| TEXAS INSTRUMENTS INCORPORATED
| Standard Linear and Logic Group
| IBIS Model of SN74CBT3383
| 10-BIT FET BUS-EXCHANGE SWITCHES
| This file contains package information for the following:
|  SSOP 24-pin (DB) package as [Component] CBT3383_DB
|  SSOP 24-pin (DBQ) package as [Component] CBT3383_DBQ
|  TVSOP 24-pin (DGV) package as [Component] CBT3383_DGV
|  SOIC 24-pin (DW) package as [Component] CBT3383_DW
|  TSSOP 24-pin (PW) package as [Component] CBT3383_PW
| This device can be powered at the following Vccs:
|  5 volt Vcc
| This file provides unique models under the [Model Selector] for each Vcc.
| For operation at a specific Vcc, select the appropriate model after each
| [Model Selector] keyword.
[IBIS Ver]   3.2
[Comment char]  |_char
[File Name]   sn74cbt3383.ibs
[File Rev]   1.1 | e_die
[Date]   April 17, 2003
[Source]   Data created from TI-SPICE simulations at TI-SLL.
[Notes]   The following is an IBIS list for the CBT3383.
   Please contact sllibis@ti.com with questions and
   comments concerning SLL IBIS models.
   - Power-clamp data has been deleted since there is no
   power-clamp diode in the device.
   - Non-monotonic data due to device characteristics.
[Disclaimer] Property of Texas Instruments Incorporated.  Unauthorized
   reproduction and/or distribution is strictly prohibited.
   This product is protected under copyright law.
   Created  2003, (C) Copyright  2003, Texas Instruments
   Incorporated, All Rights Reserved
   UNLESS THERE IS A SIGNED, WRITTEN AGREEMENT TO THE
   CONTRARY, TEXAS INSTRUMENTS (TI) IS PROVIDING THE IBIS
   MODELS  AND WITHOUT ANY WARRANTY, EXPRESSED OR
   IMPLIED.  TI assumes no liability for:
   1) the accuracy of the IBIS models provided to your
   company;
   2) the proper functioning of these IBIS Models in your
   design or for any resulting applications; or
   3) infringement of patents, copyrights or intellectual
   property rights resulting from your use of these IBIS
   models.
   TI provides IBIS Models as a service to our customers.
   You and your company shall not distribute, sell or give
   these models to anyone else without prior written
   permission from TI.
   TI reserves the right to make changes to our products or
   to discontinue any semiconductor product or service
   without notice, and advises our customers to obtain the
   latest version of relevant information to verify, before
   placing orders, that the information being relied on is
   current.
   Please be aware that your receipt and use of the IBIS
   information provided shall serve as acceptance of these
   terms and conditions.  If you do not accept these terms,
   you should return or destroy the IBIS models and any
   other accompanying information immediately.
| Component CBT3383_DB 24-pin SSOP
[Component]   CBT3383_DB
[Manufacturer]   Texas Instruments, Inc.
[Package]
|   typ   min   max
R_pkg   4.500e-02   4.000e-02   4.900e-02
L_pkg   3.668e-09   3.226e-09   4.415e-09
C_pkg   4.160e-13   3.490e-13   5.070e-13
[Pin]   signal_name   model_name   R_pin   L_pin   C_pin
1   NBE   CBT3383E_NBE   4.200e-02   4.299e-09   5.030e-13
2   1B1   CBT3383E_IO   4.000e-02   3.960e-09   4.990e-13
3   1A1   CBT3383E_IO   4.200e-02   3.775e-09   4.170e-13
4   1A2   CBT3383E_IO   4.700e-02   3.487e-09   3.690e-13
5   1B2   CBT3383E_IO   4.600e-02   3.347e-09   3.520e-13
6   2B1   CBT3383E_IO   4.900e-02   3.352e-09   3.710e-13
7   2A1   CBT3383E_IO   4.600e-02   3.226e-09   3.630e-13
8   2A2   CBT3383E_IO   4.700e-02   3.289e-09   3.490e-13
9   2B2   CBT3383E_IO   4.700e-02   3.347e-09   3.610e-13
10   3B1   CBT3383E_IO   4.100e-02   3.576e-09   4.090e-13
11   3A1   CBT3383E_IO   4.100e-02   3.995e-09   5.030e-13
12   GND   GND   4.500e-02   4.415e-09   5.070e-13
13   BX   CBT3383E_BX   4.300e-02   4.337e-09   5.060e-13
14   3A2   CBT3383E_IO   4.200e-02   4.003e-09   5.040e-13
15   3B2   CBT3383E_IO   4.100e-02   3.686e-09   4.100e-13
16   4B1   CBT3383E_IO   4.800e-02   3.355e-09   3.490e-13
17   4A1   CBT3383E_IO   4.700e-02   3.301e-09   3.530e-13
18   4A2   CBT3383E_IO   4.800e-02   3.268e-09   3.660e-13
19   4B2   CBT3383E_IO   4.800e-02   3.269e-09   3.660e-13
20   5B1   CBT3383E_IO   4.700e-02   3.314e-09   3.490e-13
21   5A1   CBT3383E_IO   4.800e-02   3.399e-09   3.550e-13
22   5A2   CBT3383E_IO   4.100e-02   3.688e-09   4.120e-13
23   5B2   CBT3383E_IO   4.200e-02   4.003e-09   5.040e-13
24   VCC   POWER   4.300e-02   4.347e-09   5.050e-13
| Component CBT3383_DBQ 24-pin SSOP
[Component]   CBT3383_DBQ
[Manufacturer]   Texas Instruments, Inc.
[Package]
|   typ   min   max
R_pkg   4.400e-02   3.100e-02   6.600e-02
L_pkg   3.074e-09   2.348e-09   4.044e-09
C_pkg   3.220e-13   2.340e-13   4.460e-13
[Pin]   signal_name   model_name   R_pin   L_pin   C_pin
1   NBE   CBT3383E_NBE   6.500e-02   4.044e-09   4.290e-13
2   1B1   CBT3383E_IO   6.600e-02   3.824e-09   4.460e-13
3   1A1   CBT3383E_IO   3.100e-02   3.011e-09   3.210e-13
4   1A2   CBT3383E_IO   3.200e-02   2.699e-09   2.590e-13
5   1B2   CBT3383E_IO   3.500e-02   2.519e-09   2.450e-13
6   2B1   CBT3383E_IO   3.500e-02   2.348e-09   2.340e-13
7   2A1   CBT3383E_IO   3.500e-02   2.348e-09   2.340e-13
8   2A2   CBT3383E_IO   3.500e-02   2.518e-09   2.450e-13
9   2B2   CBT3383E_IO   3.200e-02   2.699e-09   2.590e-13
10   3B1   CBT3383E_IO   3.100e-02   3.011e-09   3.210e-13
11   3A1   CBT3383E_IO   6.600e-02   3.824e-09   4.460e-13
12   GND   GND   6.500e-02   4.044e-09   4.290e-13
13   BX   CBT3383E_BX   6.500e-02   4.044e-09   4.290e-13
14   3A2   CBT3383E_IO   6.600e-02   3.824e-09   4.460e-13
15   3B2   CBT3383E_IO   3.100e-02   3.011e-09   3.210e-13
16   4B1   CBT3383E_IO   3.200e-02   2.699e-09   2.590e-13
17   4A1   CBT3383E_IO   3.500e-02   2.518e-09   2.450e-13
18   4A2   CBT3383E_IO   3.500e-02   2.348e-09   2.340e-13
19   4B2   CBT3383E_IO   3.500e-02   2.348e-09   2.340e-13
20   5B1   CBT3383E_IO   3.500e-02   2.518e-09   2.450e-13
21   5A1   CBT3383E_IO   3.200e-02   2.699e-09   2.590e-13
22   5A2   CBT3383E_IO   3.100e-02   3.011e-09   3.210e-13
23   5B2   CBT3383E_IO   6.600e-02   3.824e-09   4.460e-13
24   VCC   POWER   6.500e-02   4.044e-09   4.290e-13
| Component CBT3383_DGV 24-pin TVSOP
[Component]   CBT3383_DGV
[Manufacturer]   Texas Instruments, Inc.
[Package]
|   typ   min   max
R_pkg   4.300e-02   3.900e-02   4.700e-02
L_pkg   2.601e-09   2.312e-09   3.626e-09
C_pkg   3.580e-13   2.770e-13   5.950e-13
[Pin]   signal_name   model_name   R_pin   L_pin   C_pin
1   NBE   CBT3383E_NBE   4.300e-02   3.625e-09   5.950e-13
2   1B1   CBT3383E_IO   4.000e-02   2.656e-09   4.020e-13
3   1A1   CBT3383E_IO   3.900e-02   2.338e-09   3.080e-13
4   1A2   CBT3383E_IO   4.600e-02   2.354e-09   2.770e-13
5   1B2   CBT3383E_IO   4.500e-02   2.312e-09   2.850e-13
6   2B1   CBT3383E_IO   4.700e-02   2.318e-09   2.820e-13
7   2A1   CBT3383E_IO   4.700e-02   2.318e-09   2.820e-13
8   2A2   CBT3383E_IO   4.500e-02   2.312e-09   2.850e-13
9   2B2   CBT3383E_IO   4.600e-02   2.353e-09   2.780e-13
10   3B1   CBT3383E_IO   3.900e-02   2.338e-09   3.080e-13
11   3A1   CBT3383E_IO   4.100e-02   2.660e-09   4.020e-13
12   GND   GND   4.300e-02   3.625e-09   5.950e-13
13   BX   CBT3383E_BX   4.400e-02   3.626e-09   5.940e-13
14   3A2   CBT3383E_IO   4.000e-02   2.658e-09   4.020e-13
15   3B2   CBT3383E_IO   3.900e-02   2.343e-09   3.110e-13
16   4B1   CBT3383E_IO   4.600e-02   2.353e-09   2.780e-13
17   4A1   CBT3383E_IO   4.500e-02   2.312e-09   2.850e-13
18   4A2   CBT3383E_IO   4.700e-02   2.319e-09   2.820e-13
19   4B2   CBT3383E_IO   4.700e-02   2.319e-09   2.820e-13
20   5B1   CBT3383E_IO   4.500e-02   2.312e-09   2.850e-13
21   5A1   CBT3383E_IO   4.600e-02   2.353e-09   2.780e-13
22   5A2   CBT3383E_IO   3.900e-02   2.337e-09   3.080e-13
23   5B2   CBT3383E_IO   4.000e-02   2.658e-09   4.020e-13
24   VCC   POWER   4.400e-02   3.626e-09   5.950e-13
| Component CBT3383_DW 24-pin SOIC
[Component]   CBT3383_DW
[Manufacturer]   Texas Instruments, Inc.
[Package]
|   typ   min   max
R_pkg   3.700e-02   3.000e-02   4.700e-02
L_pkg   5.146e-09   3.993e-09   6.885e-09
C_pkg   7.580e-13   5.120e-13   1.067e-12
[Pin]   signal_name   model_name   R_pin   L_pin   C_pin
1   NBE   CBT3383E_NBE   3.900e-02   6.885e-09   1.067e-12
2   1B1   CBT3383E_IO   4.200e-02   5.950e-09   9.580e-13
3   1A1   CBT3383E_IO   4.700e-02   5.317e-09   7.910e-13
4   1A2   CBT3383E_IO   3.100e-02   4.651e-09   6.110e-13
5   1B2   CBT3383E_IO   3.000e-02   3.993e-09   5.120e-13
6   2B1   CBT3383E_IO   3.000e-02   4.083e-09   6.110e-13
7   2A1   CBT3383E_IO   3.000e-02   4.083e-09   6.110e-13
8   2A2   CBT3383E_IO   3.000e-02   3.993e-09   5.120e-13
9   2B2   CBT3383E_IO   3.100e-02   4.652e-09   6.110e-13
10   3B1   CBT3383E_IO   4.700e-02   5.317e-09   7.910e-13
11   3A1   CBT3383E_IO   4.200e-02   5.950e-09   9.590e-13
12   GND   GND   3.900e-02   6.885e-09   1.067e-12
13   BX   CBT3383E_BX   3.900e-02   6.885e-09   1.067e-12
14   3A2   CBT3383E_IO   4.200e-02   5.950e-09   9.590e-13
15   3B2   CBT3383E_IO   4.700e-02   5.317e-09   7.910e-13
16   4B1   CBT3383E_IO   3.100e-02   4.652e-09   6.110e-13
17   4A1   CBT3383E_IO   3.000e-02   3.993e-09   5.120e-13
18   4A2   CBT3383E_IO   3.000e-02   4.083e-09   6.100e-13
19   4B2   CBT3383E_IO   3.000e-02   4.083e-09   6.100e-13
20   5B1   CBT3383E_IO   3.000e-02   3.993e-09   5.120e-13
21   5A1   CBT3383E_IO   3.100e-02   4.651e-09   6.110e-13
22   5A2   CBT3383E_IO   4.700e-02   5.317e-09   7.910e-13
23   5B2   CBT3383E_IO   4.200e-02   5.950e-09   9.580e-13
24   VCC   POWER   3.900e-02   6.885e-09   1.067e-12
| Component CBT3383_PW 24-pin TSSOP
[Component]   CBT3383_PW
[Manufacturer]   Texas Instruments, Inc.
[Package]
|   typ   min   max
R_pkg   3.900e-02   3.000e-02   4.600e-02
L_pkg   2.685e-09   2.367e-09   3.177e-09
C_pkg   3.200e-13   2.520e-13   4.340e-13
[Pin]   signal_name   model_name   R_pin   L_pin   C_pin
1   NBE   CBT3383E_NBE   3.700e-02   3.153e-09   4.340e-13
2   1B1   CBT3383E_IO   3.400e-02   2.629e-09   3.410e-13
3   1A1   CBT3383E_IO   3.200e-02   2.860e-09   3.470e-13
4   1A2   CBT3383E_IO   4.200e-02   2.741e-09   2.900e-13
5   1B2   CBT3383E_IO   4.600e-02   2.600e-09   2.620e-13
6   2B1   CBT3383E_IO   4.300e-02   2.414e-09   2.660e-13
7   2A1   CBT3383E_IO   4.200e-02   2.367e-09   2.620e-13
8   2A2   CBT3383E_IO   4.400e-02   2.461e-09   2.520e-13
9   2B2   CBT3383E_IO   4.200e-02   2.543e-09   2.740e-13
10   3B1   CBT3383E_IO   3.000e-02   2.616e-09   3.320e-13
11   3A1   CBT3383E_IO   3.700e-02   2.670e-09   3.460e-13
12   GND   GND   3.900e-02   3.177e-09   4.330e-13
13   BX   CBT3383E_BX   3.700e-02   3.111e-09   4.310e-13
14   3A2   CBT3383E_IO   3.700e-02   2.656e-09   3.450e-13
15   3B2   CBT3383E_IO   3.100e-02   2.739e-09   3.400e-13
16   4B1   CBT3383E_IO   4.200e-02   2.649e-09   2.820e-13
17   4A1   CBT3383E_IO   4.600e-02   2.532e-09   2.570e-13
18   4A2   CBT3383E_IO   4.400e-02   2.425e-09   2.660e-13
19   4B2   CBT3383E_IO   4.400e-02   2.425e-09   2.660e-13
20   5B1   CBT3383E_IO   4.600e-02   2.532e-09   2.570e-13
21   5A1   CBT3383E_IO   4.200e-02   2.648e-09   2.820e-13
22   5A2   CBT3383E_IO   3.100e-02   2.738e-09   3.390e-13
23   5B2   CBT3383E_IO   3.600e-02   2.653e-09   3.440e-13
24   VCC   POWER   3.700e-02   3.110e-09   4.310e-13
[Series Switch Groups]
| Function Group States
On  1 /   | 1A1-5A1->1B1-5B1,1A2-5A2->1B2-5B2 NBE LOW, BX LOW
On  2 /   | 1A1-5A1->1B2-5B2,1A2-5A2->1B1-5B1 NBE LOW, BX HIGH
Off 1 2 /   | DISABLE ALL, NBE HIGH
[Series Pin Mapping]   pin_2   model_name   function_table_group
|1A1-5A1-->1B1-5B1
3   2   CBT3383E_IO_S   1
7   6   CBT3383E_IO_S   1
11   10   CBT3383E_IO_S   1
17   16   CBT3383E_IO_S   1
21   20   CBT3383E_IO_S   1
|1A2-5A2-->1B2-5B2
4   5   CBT3383E_IO_S   1
8   9   CBT3383E_IO_S   1
14   15   CBT3383E_IO_S   1
18   19   CBT3383E_IO_S   1
22   23   CBT3383E_IO_S   1
|1A1-5A1-->1B2-5B2
3   5   CBT3383E_IO_S   2
7   9   CBT3383E_IO_S   2
11   15   CBT3383E_IO_S   2
17   19   CBT3383E_IO_S   2
21   23   CBT3383E_IO_S   2
|1A2-5A2-->1B1-5B1
4   2   CBT3383E_IO_S   2
8   6   CBT3383E_IO_S   2
14   10   CBT3383E_IO_S   2
18   16   CBT3383E_IO_S   2
22   20   CBT3383E_IO_S   2
[Model]   CBT3383E_IO_S
Model_type  Series_switch
| variable   typ   min   max
C_comp   0   0   0
[Temperature Range]   40   100   -40
| Ambient temperature   25   85   -40
[Voltage range]   5   4.5   5.5
[On]
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[Off]
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| Models and submodels in the file (4): CBT3383E_NBE (Input), CBT3383E_BX (Input), CBT3383E_IO_S (Series_switch), CBT3383E_IO (Terminator)
